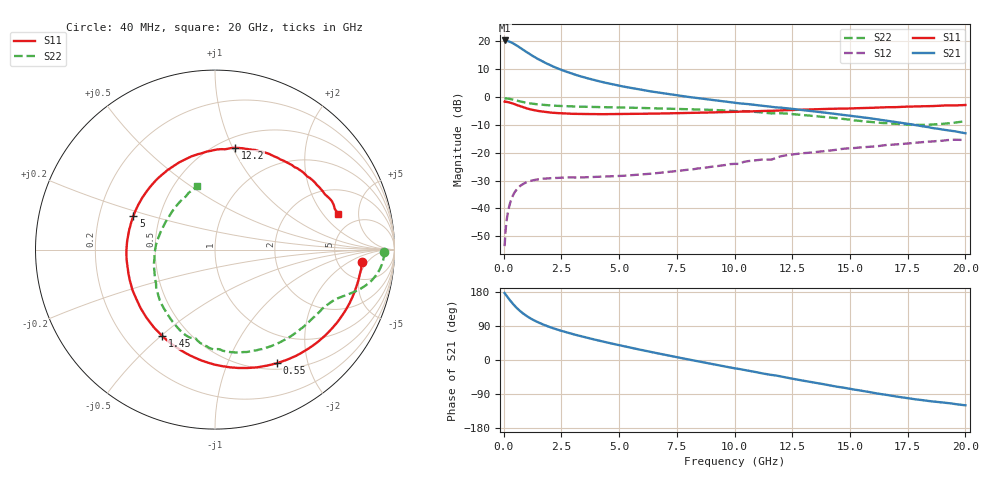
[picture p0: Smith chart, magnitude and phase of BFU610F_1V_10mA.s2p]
! Filename:  P:\Prog\Test\Noise\ATS_data\Testdata_Net\SplitFiles\BFU610_2W_A5_HighFreq_1V_10mA_D.s2p
! Date/Time: Wed 10/Aug/2011 16:55:00
! BFU610_2W_A5_HighFreq_1V_1mA_10mA_Bias6_R.s2p
! MDIF S-parameter v. bias file
! BFU610_2W_A5_HighFreq_1V_1mA_10mA
! Date/time Mon Aug 08 13:53:02 2011
! VAR V_out= 1.0002
! VAR I_out= 10.0000
! VAR V_in= 0.9509
! VAR I_in= 0.1066
! Device data file deembeded for feedlines and parallel
! Original file: \SplitFiles\BFU610_2W_A5_HighFreq_1V_10mA_R.s2p
! Feed-files: PR003V01_101208_Feed1.s2p, PR003V01_101208_Feed2.s2p
! Parallel-file: PR003V01_101208_Par.s2p
# MHz S MA R 50
!  Freq-MHz  S11-mag  S11-arg  S21-mag  S21-arg  S12-mag  S12-arg  S22-mag  S22-arg
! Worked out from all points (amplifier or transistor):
!   167 points, 40 MHz to 20 GHz, reference 50 ohm
!   highest |S21| = 20.2 dB at 40 MHz (marker M1)
!   |S21| within 3 dB of that: start of sweep to 781.9 MHz
!   unconditionally stable (mu >= 1): start of sweep to 53.69 MHz; 1.422 GHz to end of sweep
!   at 550 MHz: K = 0.46, MSG = 25.9 dB, |S12| = -33.3 dB
!   at 4.2 GHz: K = 2.99, MAG = 9.4 dB, |S12| = -28.6 dB
!   at 20 GHz: K = 5.51, MAG = -9.2 dB, |S12| = -15.3 dB
!   S11 on the Smith chart (normalised r, x): 40 MHz: 8.59, -3.67; 550 MHz: 0.58, -1.53; 1.45 GHz: 0.36, -0.51; 5 GHz: 0.35, +0.17; 12.2 GHz: 0.60, +1.02; 20 GHz: 3.59, +2.89
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40  0.8211 -4.9  10.28 176.8  0.002109 65.1  0.9422 -0.8
140  0.8124 -17.0  10.11 168.3  0.006616 73.8  0.9377 -4.0
220  0.7995 -26.4  9.893 161.7  0.01011 70.9  0.9277 -6.2
300  0.7832 -35.5  9.584 155.5  0.01337 67.0  0.9146 -8.3
400  0.7592 -46.4  9.153 148.2  0.01705 61.9  0.8952 -10.6
550  0.7214 -61.4  8.421 138.3  0.02151 54.5  0.8634 -13.3
750  0.6723 -78.8  7.423 127.1  0.02598 46.4  0.8236 -16.1
950  0.6313 -93.5  6.535 117.9  0.02903 40.2  0.7912 -18.1
1200  0.5923 -108.7  5.614 108.5  0.03147 34.4  0.76 -19.9
1450  0.5643 -121.3  4.88 100.7  0.0331 30.0  0.7371 -21.5
1750  0.54 -133.9  4.186 92.7  0.03424 26.4  0.7176 -23.3
2200  0.5163 -148.8  3.427 82.7  0.03513 22.5  0.6973 -26.2
2800  0.5007 -164.2  2.753 71.6  0.03605 20.1  0.6802 -29.8
3400  0.4941 -176.5  2.294 62.0  0.03595 19.5  0.6681 -34.0
5000  0.4918 157.7  1.591 39.1  0.03818 21.9  0.6463 -45.6
6800  0.5038 134.7  1.178 16.0  0.04374 26.1  0.6222 -59.8
8600  0.5222 114.4  0.9309 -5.6  0.05302 28.4  0.5921 -74.6
10200  0.5415 97.9  0.7674 -23.7  0.06292 28.6  0.5544 -88.2
12200  0.5776 78.9  0.6299 -45.6  0.08936 23.4  0.504 -109.0
13400  0.5987 68.0  0.5517 -58.9  0.1014 14.7  0.455 -123.8
16800  0.6542 39.9  0.3659 -94.3  0.1387 -8.2  0.3324 179.3
20000  0.7155 15.9  0.2231 -119.5  0.1715 -36.5  0.3659 106.0
